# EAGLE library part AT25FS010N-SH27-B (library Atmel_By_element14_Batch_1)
High Speed Small Sectored SPI Flash Memory
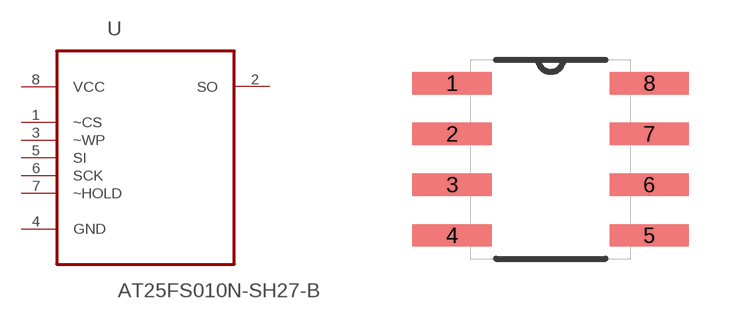
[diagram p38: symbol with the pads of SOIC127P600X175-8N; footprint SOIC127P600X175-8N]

Designator prefix U

## AT25FS010N-SH27-B (MPN: AT25FS010N-SH27-B; OC_FARNELL: 1715447; OC_NEWARK: -; PACKAGE: SOIC-8; SUPPLIER: Atmel)  [SOIC127P600X175-8N]
1  ~CS  in
2  SO  out
3  ~WP  in
4  GND  pas
5  SI  in
6  SCK  in
7  ~HOLD  in
8  VCC  pwr

## Footprint SOIC127P600X175-8N (pad centres in mm)
smd 1.981 x 0.559: 1 -2.464,1.905; 2 -2.464,0.635; 3 -2.464,-0.635; 4 -2.464,-1.905; 5 2.464,-1.905; 6 2.464,-0.635; 7 2.464,0.635; 8 2.464,1.905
